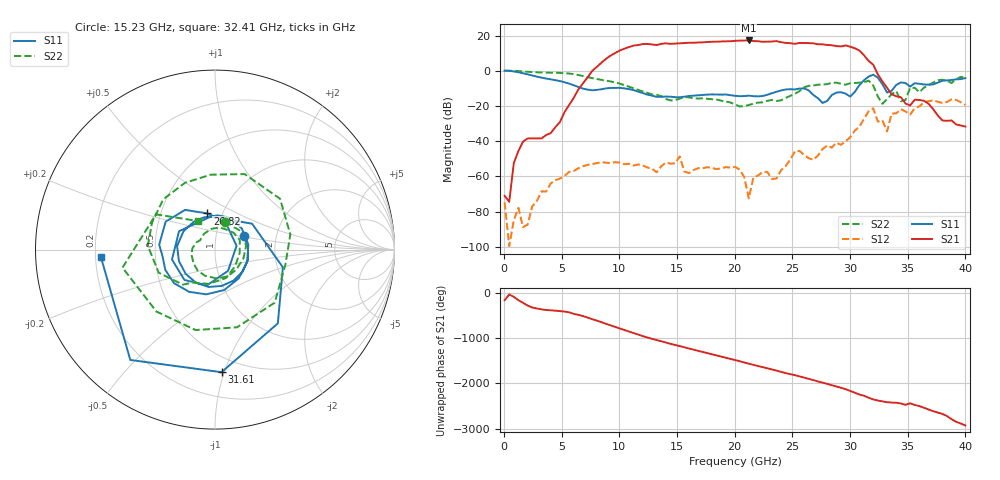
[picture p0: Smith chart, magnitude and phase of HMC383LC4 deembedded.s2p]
!Hittite Microwave Corporation
!20 Alpha Road
!Chelmsford, MA 01824
!Tel: 978-250-3343
!Fax: 978-250-3373
!Device: HMC383LC4, 12-30 GHz, GaAs PHEMT MMIC Driver Amplifier in leadless "Pb free" RoHS compliant SMT package
!Misc: Vdd = +5V, data includes two Southwest connectors, Room
# MHZ S MA R 50
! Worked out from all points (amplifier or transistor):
!   101 points, 50 MHz to 40 GHz, reference 50 ohm
!   highest |S21| = 17.2 dB at 21.22 GHz (marker M1)
!   |S21| within 3 dB of that: 11.19 GHz to 28.64 GHz (17.45 GHz wide, 87.6 % of centre)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
!   unconditionally stable (mu >= 1): 620.1 MHz to end of sweep
!   at 6.442 GHz: K = 371.97, MAG = -6.3 dB, |S12| = -55.3 dB
!   at 20.02 GHz: K = 35.90, MAG = 17.2 dB, |S12| = -54.5 dB
!   at 40 GHz: K = 64.29, MAG = -27.2 dB, |S12| = -19.4 dB
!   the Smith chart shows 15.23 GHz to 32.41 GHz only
!   S11 on the Smith chart (normalised r, x): 15.23 GHz: 1.37, +0.21; 26.82 GHz: 0.85, +0.36; 31.61 GHz: 0.38, -0.98; 32.41 GHz: 0.22, -0.03
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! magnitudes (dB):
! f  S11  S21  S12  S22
! 50 MHz  0.1  -71.0  -74.7  0.0
! 449.5 MHz  -0.1  -74.4  -99.6  0.0
! 849 MHz  -0.4  -52.4  -84.8  0.0
! 1.648 GHz  -1.4  -40.2  -88.8  -0.4
! 4.045 GHz  -4.9  -35.4  -64.0  -1.1
! 6.841 GHz  -10.1  -7.2  -54.2  -3.0
! 10.04 GHz  -9.7  11.5  -52.2  -7.3
! 13.63 GHz  -14.8  15.3  -54.2  -14.4
! 15.23 GHz  -15.0  15.6  -48.6  -15.9
! 16.03 GHz  -14.3  15.9  -58.1  -15.1
! 20.02 GHz  -14.2  17.0  -54.5  -19.1
! 21.22 GHz  -14.1  17.2  -72.4  -19.4
! 21.62 GHz  -14.4  16.9  -60.4  -18.6
! 23.62 GHz  -11.9  16.8  -61.2  -17.1
! 25.22 GHz  -10.6  15.3  -45.7  -13.1
! 26.82 GHz  -13.7  15.6  -50.5  -8.4
! 30.01 GHz  -14.7  13.7  -37.7  -7.0
! 31.61 GHz  -3.3  5.6  -23.0  -5.6
! 32.41 GHz  -3.9  -2.1  -28.9  -14.6
! 33.21 GHz  -12.4  -9.6  -34.4  -16.0
! 33.61 GHz  -11.3  -13.3  -24.3  -13.4
! 40 GHz  -4.2  -31.7  -19.4  -3.8
